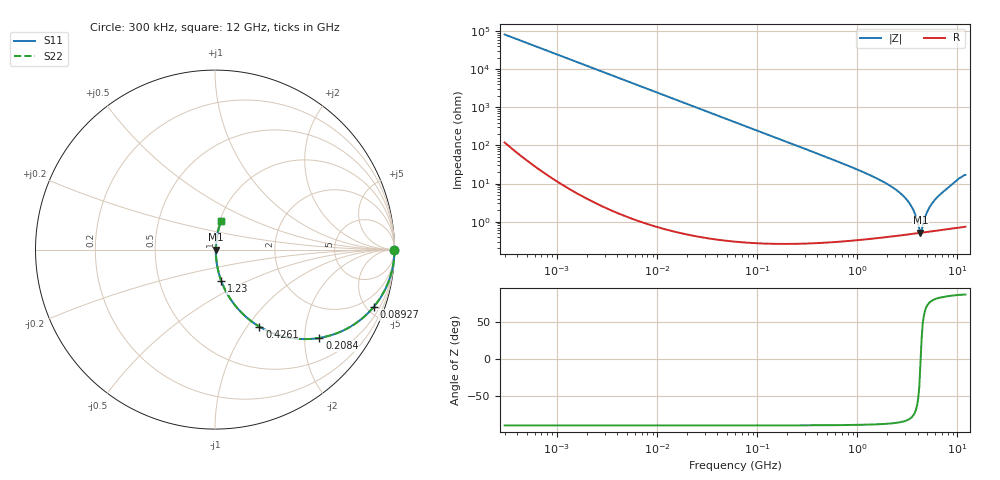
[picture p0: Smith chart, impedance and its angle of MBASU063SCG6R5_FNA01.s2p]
! MBASU063SCG6R5_FNA01  S-PARAMETER MODEL  ( General Type )
! Model Generated by TAIYO YUDEN Corporation (http://www.ty-top.com)
! Version 1.0
! TAIYO YUDEN Control No. 130801
! Copyright(c) 2013 TAIYO YUDEN CO.,LTD. All Rights Reserved.
! Product Description (link to TY-COMPAS)
! https://ds.yuden.co.jp/TYCOMPAS/or/detail?pn=MBASU063SCG6R5DFNA01&u=M
! Products Name : Multilayer Ceramic Capacitors
! Characteristics :
!  Capacitance : 6.5 pF , Rated Voltage : 50V , TCC : CG / C0G
!  Case Size : 0.6 x 0.3 / 0.024 x 0.012 [mm/inch] , Thickness : 0.3 / 0.012 [mm/inch]
!  (Conditions: Temperature = 25 degC , DC Bias Current/Voltage = 0A / 0V)
! External Node Assignments :
!  1  o---| |---o  2
! GND o---------o GND
! Frequency Range : 0.3MHz  -  12000MHz  [ 401 STEP ]
# MHz S RI R 50
! Freq[MHz].  S11 Real  S11 Imag  S21 Real  S21 Imag  S12 Real  S12 Imag  S22 Real  S22 Imag
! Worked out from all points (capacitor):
!   401 points, 300 kHz to 12 GHz, reference 50 ohm
!   read as one part in series: C = 6.46 pF near 316.3 kHz
!   lowest |Z| = 510 mohm at 4.271 GHz (marker M1)
!   series resonance near 4.284 GHz, so ESL is about 210 pH
!   S11 on the Smith chart (normalised r, x): 300 kHz: open; 89.27 MHz: 1.01, -5.52; 208.4 MHz: 1.01, -2.36; 426.1 MHz: 1.01, -1.15; 1.23 GHz: 1.01, -0.37; 12 GHz: 1.01, +0.34
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0.3  1 -0.00122  3.26e-06 0.00122  3.26e-06 0.00122  1 -0.00122
1.769972  0.9999 -0.00718  5.4e-05 0.00718  5.4e-05 0.00718  0.9999 -0.00718
10.44266  0.9982 -0.0423  0.00181 0.0423  0.00181 0.0423  0.9982 -0.0423
27.10171  0.988 -0.1087  0.012 0.1087  0.012 0.1087  0.988 -0.1087
60  0.9439 -0.2298  0.0561 0.2298  0.0561 0.2298  0.9439 -0.2298
89.27472  0.8836 -0.3202  0.1164 0.3202  0.1164 0.3202  0.8836 -0.3202
208.3979  0.5816 -0.4922  0.4184 0.4922  0.4184 0.4922  0.5816 -0.4922
353.9943  0.324 -0.4661  0.676 0.4661  0.676 0.4661  0.324 -0.4661
426.1204  0.2479 -0.4294  0.7521 0.4294  0.7521 0.4294  0.2479 -0.4294
686.4755  0.1111 -0.31  0.8889 0.31  0.8889 0.31  0.1111 -0.31
1229.528  0.0359 -0.1768  0.9641 0.1768  0.9641 0.1768  0.0359 -0.1768
2088.533  0.012 -0.0887  0.988 0.0887  0.988 0.0887  0.012 -0.0887
2722.03  0.00724 -0.0536  0.9928 0.0536  0.9928 0.0536  0.00724 -0.0536
3276.641  0.0056 -0.0312  0.9944 0.0312  0.9944 0.0312  0.0056 -0.0312
3642.919  0.00515 -0.0189  0.9948 0.0189  0.9948 0.0189  0.00515 -0.0189
4050.141  0.00502 -0.00678  0.995 0.00678  0.995 0.00678  0.00502 -0.00678
4270.516  0.00506 -0.000347  0.9949 0.000347  0.9949 0.000347  0.00506 -0.000347
4502.883  0.00519 0.00588  0.9948 -0.00588  0.9948 -0.00588  0.00519 0.00588
5140.631  0.00582 0.0204  0.9942 -0.0204  0.9942 -0.0204  0.00582 0.0204
5868.704  0.0069 0.035  0.9931 -0.035  0.9931 -0.035  0.0069 0.035
9968.853  0.0219 0.1215  0.9781 -0.1215  0.9781 -0.1215  0.0219 0.1215
12000  0.0341 0.1609  0.9659 -0.1609  0.9659 -0.1609  0.0341 0.1609
